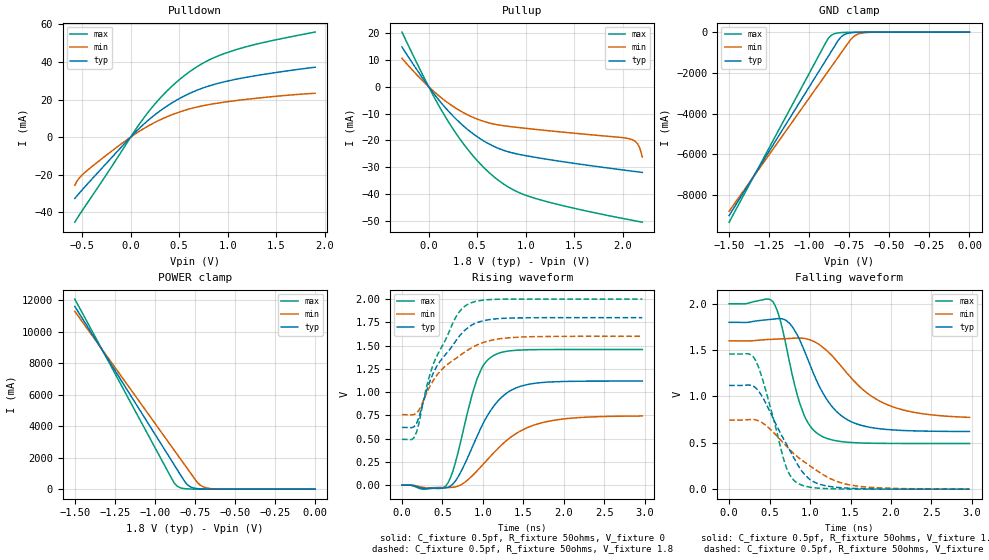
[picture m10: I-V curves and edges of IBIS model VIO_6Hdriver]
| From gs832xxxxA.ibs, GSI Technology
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|  signals   DQA1-DQA9, DQB1-DQB9, DQC1-DQC9, DQD1-DQD9
[Model]   VIO_6Hdriver
Model_type   I/O
Polarity   Non-Inverting
Vinl  =   0.54v
Vinh  =   1.08v
Vmeas =   0.9v
Cref  =   0pF
Rref  =   50
Vref  =   0.9v
|  variable   typ   min   max
C_comp   3.0pF   2.5pF   3.5pF
|  variable   typ   min   max
[Temperature Range]   50   0   100
|  variable   typ   min   max
[Voltage Range]   1.8   1.6   2.0
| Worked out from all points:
|   slope of the pulldown table from 0 to 0.27 V, typ, clamps not added: 21.3 ohm
|   slope of the pullup table from 0 to 0.27 V, typ, clamps not added: 23.3 ohm
|   GND clamp passes 1 mA (typ) near -0.58 V on its own axis
|   POWER clamp passes 1 mA (typ) near -0.61 V on its own axis
|   rising waveform, C_fixture 0.5pf, R_fixture 50ohms, V_fixture 0: 20-80 % time 403ps typ, 570ps min, 265ps max; typ from 0 V to 1.12 V
|   rising waveform, C_fixture 0.5pf, R_fixture 50ohms, V_fixture 1.8: 20-80 % time 425ps typ, 504ps min, 368ps max; typ from 0.621 V to 1.8 V
|   falling waveform, C_fixture 0.5pf, R_fixture 50ohms, V_fixture 1.8: 20-80 % time 410ps typ, 608ps min, 262ps max; typ from 1.8 V to 0.622 V
|   falling waveform, C_fixture 0.5pf, R_fixture 50ohms, V_fixture 0: 20-80 % time 404ps typ, 609ps min, 265ps max; typ from 1.12 V to 0 V
[Pulldown]
| voltage   typ   min   max
-575mV    -32.66mA   -25.61mA   -45.27mA
-525mV    -29.57mA   -21.53mA   -41.16mA
-425mV    -23.82mA   -16.78mA   -33.46mA
-100mV    -5.543mA   -3.744mA   -8.091mA
125mV     6.391mA    4.233mA    9.468mA
225mV     10.85mA    7.162mA    16.08mA
325mV     14.77mA    9.711mA    21.92mA
525mV     21.16mA    13.74mA    31.55mA
750mV     26.25mA    16.75mA    39.49mA
1V        29.85mA    18.86mA    45.1mA
1.35V     33.21mA    20.98mA    50.13mA
1.9V      37.21mA    23.34mA    55.89mA
[Pullup]
| voltage (VDDQ-Vout) typ   min   max
-275mV    14.8mA     10.56mA    20.34mA
25mV      -1.232mA   -846.9uA   -1.746mA
225mV     -9.933mA   -6.682mA   -14.29mA
350mV     -14.35mA   -9.496mA   -20.87mA
475mV     -17.99mA   -11.68mA   -26.51mA
700mV     -22.68mA   -14.11mA   -34.34mA
875mV     -24.75mA   -15mA      -38.46mA
1.075V    -26.15mA   -15.79mA   -41.33mA
2.05V     -31.22mA   -19.24mA   -49.41mA
2.15V     -31.68mA   -21.21mA   -50.1mA
2.175V    -31.8mA    -22.89mA   -50.27mA
2.2V      -31.92mA   -26.11mA   -50.44mA
[GND Clamp]
| voltage   typ   min   max
-1.5V     -9.007A    -8.796A    -9.334A
-900mV    -1.426A    -2.122A    -562.9mA
-880mV    -1.174A    -1.9A      -292.9mA
-860mV    -921.1mA   -1.678A    -142.5mA
-820mV    -416.2mA   -1.233A    -38.58mA
-800mV    -222mA     -1.011A    -23.51mA
-780mV    -116.3mA   -788.8mA   -16.2mA
-740mV    -33.04mA   -348.7mA   -9.876mA
-720mV    -18.57mA   -198.2mA   -8.142mA
-680mV    -6.87mA    -61.92mA   -5.539mA
-580mV    -1.002mA   -3.885mA   -1.438mA
0V        -394.9pA   -781.6pA   -350.3pA
[POWER Clamp]
| voltage (VDDQ-Vout) typ   min   max
-1.5V     11.62A     11.31A     12.09A
-900mV    1.877A     2.768A     763.5mA
-880mV    1.553A     2.483A     398.4mA
-860mV    1.228A     2.198A     183.4mA
-840mV    903.6mA    1.913A     83.63mA
-800mV    304.2mA    1.344A     19.44mA
-780mV    154.7mA    1.059A     10.68mA
-740mV    39.51mA    489.9mA    4.639mA
-720mV    20.32mA    274.5mA    3.532mA
-680mV    5.894mA    82.85mA    2.298mA
-580mV    568.7uA    4.201mA    684.1uA
0V        586.6pA    1.815nA    369.9pA
[Ramp]
| voltage   typ   min   max
dV/dt_r   1.53/137p   1.35/170p   1.77/112p
dV/dt_f   1.51/136p   1.31/167p   1.77/112p
R_load  =   50ohms
[Rising Waveform]
C_fixture =   0.5pf
R_fixture =   50ohms
V_fixture =   0
| Time   V(typ)   V(min)   V(max)
0s        5.267nV    13.83nV    3.451nV
540ps     -28.98mV   -25.2mV    -10.62mV
630ps     14.03mV    -22.33mV   152.5mV
750ps     181.2mV    15.28mV    559mV
930ps     528.6mV    155.9mV    1.147V
1.02ns    692mV      240.3mV    1.306V
1.14ns    856.8mV    353.3mV    1.397V
1.38ns    1.033V     537.6mV    1.447V
1.74ns    1.104V     673mV      1.457V
2.97ns    1.119V     743.5mV    1.458V
[Rising Waveform]
C_fixture =   0.5pf
R_fixture =   50ohms
V_fixture =   1.8
V_fixture_min =   1.6
V_fixture_max =   2.0
| Time   V(typ)   V(min)   V(max)
0s        620.9mV    758.2mV    492.4mV
150ps     629.3mV    758.9mV    511.5mV
210ps     725.8mV    805.1mV    666.7mV
300ps     1.004V     980mV      1.043V
390ps     1.21V      1.13V      1.307V
660ps     1.544V     1.358V     1.798V
810ps     1.688V     1.45V      1.942V
990ps     1.764V     1.529V     1.987V
1.32ns    1.795V     1.584V     1.999V
2.97ns    1.8V       1.6V       2V
[Falling Waveform]
C_fixture =   0.5pf
R_fixture =   50ohms
V_fixture =   1.8
V_fixture_min =   1.6
V_fixture_max =   2.0
| Time   V(typ)   V(min)   V(max)
0s        1.8V       1.6V       2V
540ps     1.834V     1.617V     2.024V
630ps     1.84V      1.621V     1.83V
750ps     1.785V     1.626V     1.354V
870ps     1.615V     1.631V     933.6mV
990ps     1.362V     1.614V     694.2mV
1.14ns    1.067V     1.543V     573.5mV
1.44ns    759.8mV    1.269V     508.3mV
1.89ns    649mV      937.1mV    494.2mV
2.97ns    622.2mV    774.5mV    492.6mV
[Falling Waveform]
C_fixture =   0.5pf
R_fixture =   50ohms
V_fixture =   0
| Time   V(typ)   V(min)   V(max)
0s        1.119V     745.4mV    1.458V
240ps     1.124V     750.3mV    1.461V
330ps     1.092V     747.6mV    1.384V
450ps     932.9mV    691.2mV    1.074V
690ps     514.4mV    480.4mV    274.4mV
780ps     370.6mV    399.7mV    114.3mV
870ps     230.4mV    331.7mV    53.66mV
1.08ns    65.02mV    202.3mV    12.71mV
1.5ns     9.694mV    44.33mV    942.7uV
2.97ns    34.48uV    732.2uV    671.4nV
